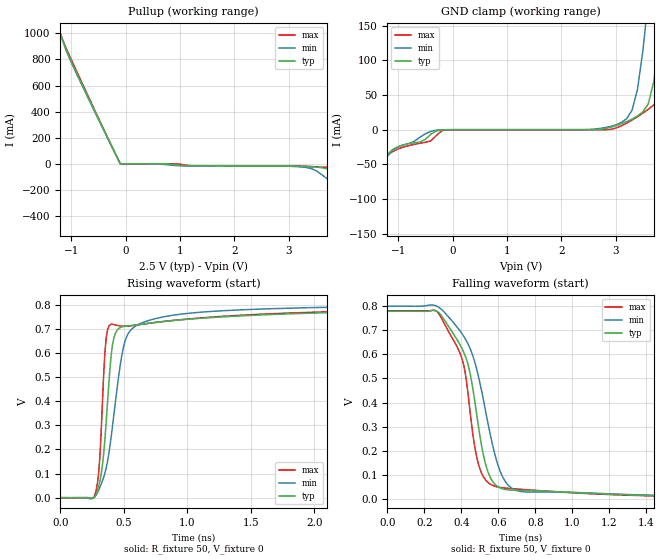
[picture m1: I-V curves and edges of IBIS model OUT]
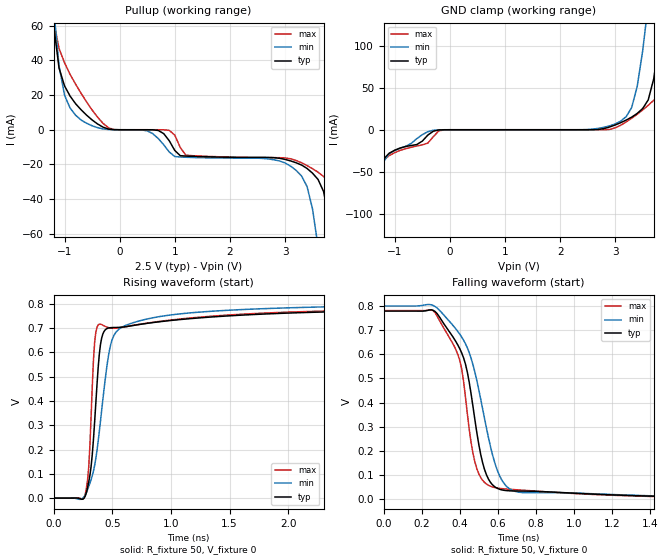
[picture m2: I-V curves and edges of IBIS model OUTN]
|   IBIS File of SG2520HHN D
|   HCSL Zdiff=100, Vcc=2.5V, fo<=212.5MHz
[IBIS Ver]   3.2
[File Name]   sg2520hhn_25v.ibs
[File Rev]   1.0
[Date]   Jan. 25, 2023
[Source]
[Notes]
Created by Minoru Kozaki
[Disclaimer]
Seiko Epson Corporation makes no warranty with respect to the
information contained herein.
[Copyright]
Copyright(C) 2023, Seiko Epson Corporation. All rights reserved.
|   Component
[Component]   SG2520HHN
[Manufacturer]  Seiko Epson Corporation
[Package]
R_pkg   17.7m   NA   NA
L_pkg   235p   NA   NA
C_pkg   208f   NA   NA
[Pin]   signal_name   model_name   R_pin   L_pin   C_pin
1   OE/ST   NC
2   NC   NC
3   GND   GND
4   OUT   OUT   17.7m   235p   208f
5   OUTN   OUTN   10.4m   129p   221f
6   VCC   POWER
[Diff Pin] inv_pin  vdiff  tdelay_typ
4   5   0   0
| Models and submodels in the file (2): OUT (Open_source), OUTN (Open_source)
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|   Model OUT
[Model]   OUT
Model_type   Open_source
Polarity   Non-Inverting
Vref = 0
Vmeas = 0.4
Rref = 50
Cref = 0
C_comp   12.0p   12.0p   12.0p
[Temperature Range]   25   105   -40
[Voltage Range]   2.5   2.25   2.75
[Pullup Reference]   2.5   2.25   2.75
[GND Clamp Reference]   0   0   0
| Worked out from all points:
|   GND clamp passes 1 mA (typ) near -0.25 V on its own axis
|   falling waveform, R_fixture 50, V_fixture 0: 20-80 % time 123ps typ, 152ps min, 107ps max; typ from 0.779 V to 0 V
|   rising waveform, R_fixture 50, V_fixture 0: 20-80 % time 72.2ps typ, 130ps min, 45ps max; typ from 0 V to 0.778 V
[Pullup]
-2.5V     3.371A     3.276A     3.476A
-1.3V     1.138A     1.157A     1.132A
-1.2V     987.8mA    998mA      992.3mA
-1.1V     877.7mA    875.8mA    890.7mA
-1V       784.2mA    777.5mA    798mA
-100mV    31.36uA    14.22uA    89.27uA
1V        -12.43mA   -15.66mA   -3.28mA
2.9V      -16.65mA   -18.23mA   -16.26mA
3.4V      -22.67mA   -35.03mA   -21.13mA
3.7V      -38.9mA    -113mA     -27.79mA
4V        -130.5mA   -205.5mA   -48.61mA
5V        -473.8mA   -515mA     -419.8mA
[GND Clamp]
-2.5V     -393mA     -369.8mA   -420.3mA
-1.7V     -165.8mA   -161.7mA   -172.8mA
-1.6V     -137.5mA   -135.8mA   -141.9mA
-1.2V     -35.69mA   -38.74mA   -37.05mA
-400mV    -6.513mA   -2.4mA     -16.1mA
3.1V      8.47mA     10.34mA    5.39mA
3.3V      15.16mA    27.81mA    13.85mA
3.6V      37.26mA    188.1mA    29.48mA
3.8V      131mA      345.9mA    43.2mA
3.9V      212.3mA    425.5mA    55.77mA
4.1V      382.8mA    585.7mA    161.6mA
5V        1.177A     1.402A     1.001A
[Falling Waveform]
R_fixture = 50
V_fixture = 0
V_fixture_min = 0
V_fixture_max = 0
0s        779.4mV    800.4mV    781.3mV
260ps     782.4mV    803.2mV    782.2mV
400ps     630.1mV    690.5mV    590.4mV
450ps     511.9mV    620mV      343.2mV
480ps     366.8mV    548mV      184.4mV
510ps     218.1mV    446.7mV    105.7mV
550ps     99.79mV    291.2mV    64.24mV
610ps     45.09mV    114mV      47.12mV
710ps     35.02mV    31.99mV    39.9mV
4ns       425uV      654uV      318uV
[Rising Waveform]
R_fixture = 50
V_fixture = 0
V_fixture_min = 0
V_fixture_max = 0
0s        153uV      237uV      126uV
280ps     11.04mV    10.5mV     27.21mV
310ps     67.32mV    42.27mV    162.3mV
340ps     178mV      83.78mV    504.4mV
360ps     310.9mV    121.8mV    659.3mV
400ps     591.2mV    253.2mV    718.8mV
440ps     688.7mV    426.4mV    715.1mV
510ps     710.7mV    650.3mV    710.4mV
710ps     723.9mV    736.6mV    723.8mV
4ns       778.1mV    798.9mV    780.4mV
[Ramp]
R_load = 50
dV/dt_r   0.47534/74.11p   0.48804/135.14p   0.47705/45.78p
dV/dt_f   0.47534/128.65p   0.48804/157.38p   0.47705/113.04p
|   Model OUTN
[Model]   OUTN
Model_type   Open_source
Polarity   Inverting
Vref = 0
Vmeas = 0.4
Rref = 50
Cref = 0
C_comp   12.0p   12.0p   12.0p
[Temperature Range]   25   105   -40
[Voltage Range]   2.5   2.25   2.75
[Pullup Reference]   2.5   2.25   2.75
[GND Clamp Reference]   0   0   0
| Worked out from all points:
|   GND clamp passes 1 mA (typ) near -0.25 V on its own axis
|   falling waveform, R_fixture 50, V_fixture 0: 20-80 % time 119ps typ, 149ps min, 103ps max; typ from 0.779 V to 0 V
|   rising waveform, R_fixture 50, V_fixture 0: 20-80 % time 72ps typ, 131ps min, 44.7ps max; typ from 0 V to 0.777 V
[Pullup]
-2.5V     901mA      871.9mA    935.9mA
-1.2V     60.69mA    70.89mA    63.14mA
-1V       25.25mA    19.88mA    38.54mA
-600mV    8.395mA    3.722mA    16.02mA
-200mV    362.5uA    113.9uA    1.078mA
900mV     -6.341mA   -12.8mA    -382uA
1.2V      -15.17mA   -15.85mA   -14.62mA
3.2V      -19.01mA   -23.34mA   -17.68mA
3.6V      -28.63mA   -67.4mA    -24.45mA
3.9V      -76.62mA   -140.9mA   -34.37mA
4.1V      -129.9mA   -190mA     -62.45mA
5V        -369.8mA   -411.3mA   -320mA
[GND Clamp]
-2.5V     -368.4mA   -348.8mA   -391.7mA
-1.6V     -128.8mA   -128mA     -132.2mA
-1.2V     -34.69mA   -37.54mA   -36.04mA
-400mV    -6.375mA   -2.378mA   -15.91mA
-100mV    -21.28uA   -12.91uA   -96.72uA
3.1V      8.395mA    10.26mA    5.333mA
3.3V      15mA       26.54mA    13.66mA
3.6V      35.53mA    149.8mA    29.02mA
3.8V      106.5mA    273.2mA    42.36mA
3.9V      166mA      335.4mA    53.04mA
4.1V      296.9mA    460.5mA    128.6mA
5V        901mA      1.036A     756mA
[Falling Waveform]
R_fixture = 50
V_fixture = 0
V_fixture_min = 0
V_fixture_max = 0
0s        778.5mV    799.4mV    780.4mV
260ps     781.6mV    801.6mV    780.1mV
400ps     622.7mV    683.1mV    574.3mV
430ps     558.9mV    643.2mV    422.3mV
460ps     433.6mV    582.2mV    232.3mV
500ps     227.1mV    453.4mV    106mV
540ps     102.3mV    295.8mV    63.63mV
600ps     44.79mV    115mV      46.65mV
700ps     34.71mV    31.44mV    39.75mV
4ns       417uV      640uV      311uV
[Rising Waveform]
R_fixture = 50
V_fixture = 0
V_fixture_min = 0
V_fixture_max = 0
0s        143uV      238uV      123uV
270ps     8.458mV    12.6mV     15.3mV
300ps     66.87mV    48.06mV    129.8mV
330ps     179.3mV    92.35mV    459.6mV
350ps     313.3mV    134.3mV    640.8mV
390ps     593mV      274.3mV    716.7mV
430ps     686.4mV    447.5mV    709.7mV
500ps     702.6mV    653.8mV    699.8mV
690ps     712mV      724.2mV    712.7mV
4ns       777mV      797.6mV    779.3mV
[Ramp]
R_load = 50
dV/dt_r   0.47523/74.07p   0.48792/137.69p   0.47690/45.33p
dV/dt_f   0.47523/125.09p   0.48792/154.59p   0.47690/109.10p
